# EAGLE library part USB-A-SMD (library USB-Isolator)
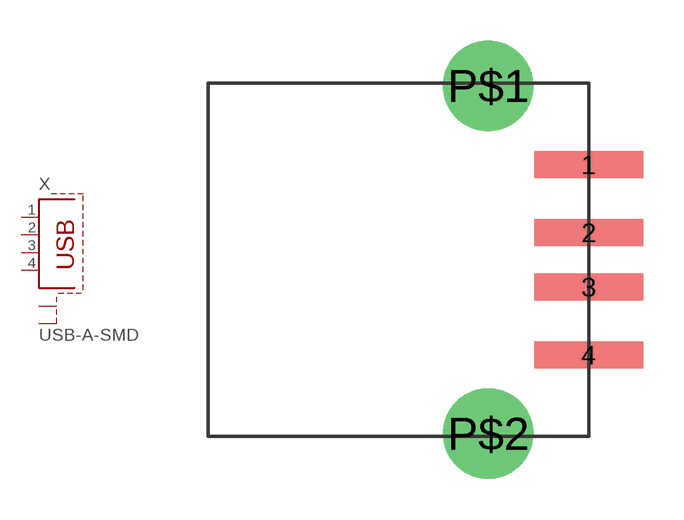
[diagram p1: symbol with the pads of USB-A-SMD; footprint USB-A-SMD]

Designator prefix X

## USB-A-SMD  [USB-A-SMD]
1  1  pas
2  2  pas
3  3  pas
4  4  pas
P$1  S1  pas
P$2  S2  pas

## Footprint USB-A-SMD (pad centres in mm)
smd 4 x 1: 1 0,3.5; 2 0,1; 3 0,-1; 4 0,-3.5
drill 2.3 pad 2.9: P$1 -3.7,6.4; P$2 -3.7,-6.4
